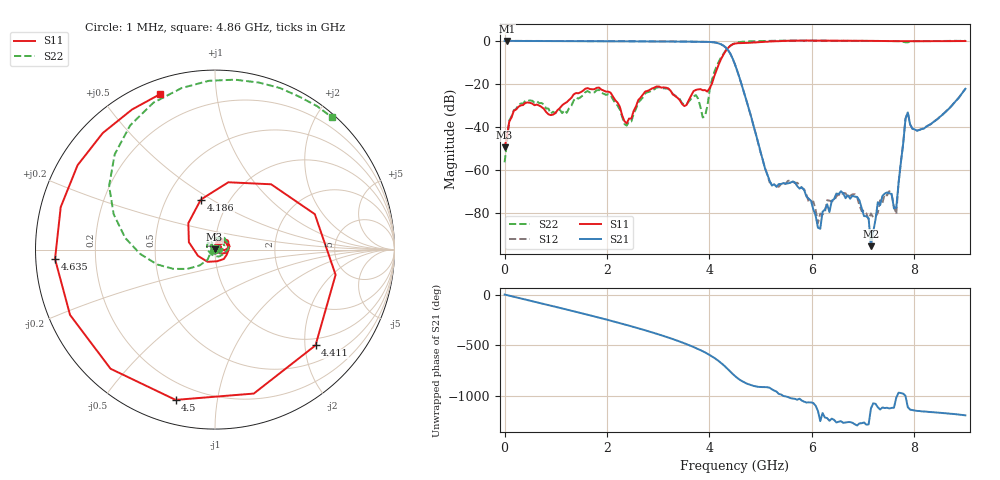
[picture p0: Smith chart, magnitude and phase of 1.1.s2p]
!Prosund Technologies,SP809B,SP82221046,V.03.04.C
!Date: Sunday, January 19, 2025 15:10:49
!Correction: S11(C  2-Port  )
!S21(C  2-Port  )
!S12(C  2-Port  )
!S22(C  2-Port  )
!S2P File: Measurement: :
# Hz S  dB  R 50
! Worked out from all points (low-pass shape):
!   201 points, 1 MHz to 9 GHz, reference 50 ohm
!   highest |S21| = 0.01 dB at 45.99 MHz (marker M1); lowest = -95.5 dB at 7.155 GHz (marker M2)
!   |S21| within 3 dB of the highest: start of sweep to 4.316 GHz
!   lowest |S11| = -49.5 dB at 1 MHz (marker M3), VSWR 1.01, Z = 49.8 + j0.225 ohm
!   |S11| at or under -10 dB: start of sweep to 4.2 GHz
!   |S22| runs from -56.5 to 0.2 dB; largest |S21 - S12| = 0.016
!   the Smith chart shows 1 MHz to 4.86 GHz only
!   S11 on the Smith chart (normalised r, x): 1 MHz: 1.00, +0.00; 4.186 GHz: 0.74, +0.45; 4.411 GHz: 0.84, -2.23; 4.5 GHz: 0.11, -0.77; 4.635 GHz: 0.06, -0.03; 4.86 GHz: 0.06, +0.71
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1000000  -49.48 137.8  -0.03 -0.1  -0.03 -0.1  -56.45 137.4
4.5995e7  -44.70 98.0  0.01 -5.8  0.04 -5.6  -47.60 94.5
2.7097e8  -30.64 45.2  -0.03 -32.9  0.00 -32.6  -29.71 33.6
7.65915e8  -31.54 12.0  -0.07 -92.9  -0.03 -92.5  -29.48 -38.5
1.53083e9  -23.21 42.2  -0.14 172.3  -0.11 172.8  -25.29 90.7
2.25075e9  -30.58 -39.7  -0.17 78.1  -0.15 78.7  -31.96 -8.0
3.015665e9  -21.21 32.3  -0.26 -33.9  -0.24 -33.3  -21.59 47.8
3.42062e9  -27.51 2.0  -0.31 -103.6  -0.28 -102.8  -27.04 -61.6
3.78058e9  -22.55 16.0  -0.41 -177.6  -0.39 -176.7  -26.90 129.6
3.915565e9  -22.87 -46.6  -0.43 149.2  -0.41 149.9  -34.95 175.0
4.185535e9  -10.76 105.9  -1.21 63.0  -1.19 63.8  -9.56 -165.6
4.41051e9  -2.23 -43.6  -6.00 -40.3  -6.01 -39.6  -2.26 136.5
4.5005e9  -1.25 -104.7  -10.98 -83.5  -10.97 -83.0  -1.04 112.8
4.635485e9  -0.98 -176.6  -20.78 -133.0  -20.80 -132.1  -0.42 83.3
4.86046e9  -0.74 109.4  -39.29 179.4  -39.34 -179.5  -0.14 48.5
5.175425e9  -0.29 51.0  -64.90 161.0  -65.70 160.2  0.07 13.3
6.03033e9  0.16 -31.5  -78.35 9.9  -74.68 -0.8  0.15 -54.1
7.155205e9  0.00 -104.2  -95.45 -43.1  -80.25 94.7  -0.01 -123.9
7.515165e9  -0.09 -122.0  -70.89 -43.2  -69.85 -40.0  -0.08 -141.6
7.65015e9  -0.10 -128.7  -77.41 63.5  -80.57 66.4  -0.09 -148.3
7.875125e9  -0.14 -138.8  -33.25 -30.6  -33.20 -29.3  -0.66 -155.3
9e9  -0.06 171.2  -22.29 -111.3  -22.31 -110.6  0.07 154.6
